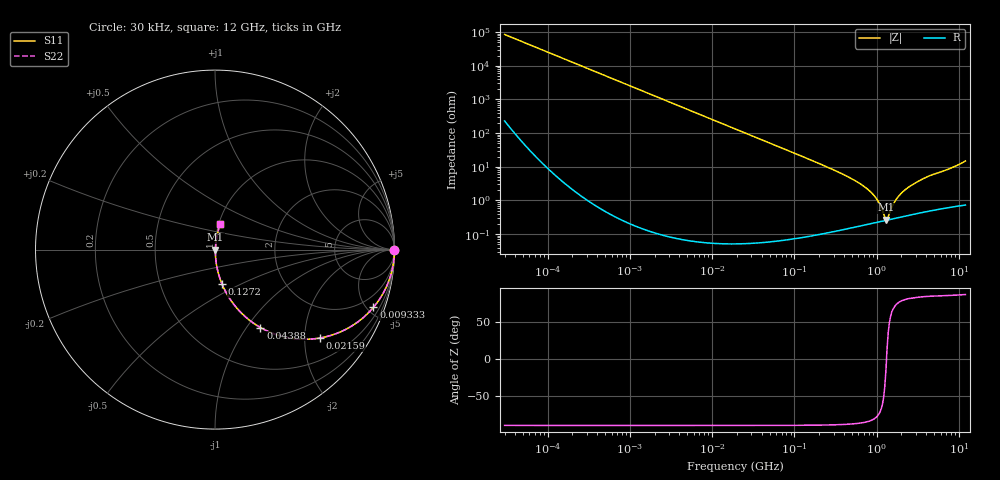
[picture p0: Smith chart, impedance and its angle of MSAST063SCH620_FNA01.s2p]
! MSAST063SCH620_FNA01  S-PARAMETER MODEL  ( Standard Model )
! Model Generated by TAIYO YUDEN Corporation (http://www.ty-top.com)
! Version 1.0
! TAIYO YUDEN Control No. 241122
! Copyright(c) 2024 TAIYO YUDEN CO.,LTD. All Rights Reserved.
! Product Description (link to TY-COMPAS)
! https://ds.yuden.co.jp/TYCOMPAS/or/detail?pn=MSAST063SCH620JFNA01&u=M
! Products Name : Multilayer Ceramic Capacitors
! Characteristics :
!  Capacitance : 62 [pF] , Rated Voltage : 25 [V] , TCC : CH / C0H
!  Case Size : 0.6 x 0.3 / 0.024 x 0.012 [mm/inch] , Thickness : 0.3 / 0.012 [mm/inch]
!  (Conditions: Temperature = 25 [degC] , DC Bias Voltage = 0 [V])
! External Node Assignments :
!  1  o---| |---o  2
! GND o---------o GND
! Frequency Range : 0.03MHz  -  12000MHz  [ 401 STEP ]
# MHZ S RI R 50
! Freq[MHz].  S11 Real  S11 Imag  S21 Real  S21 Imag  S12 Real  S12 Imag  S22 Real  S22 Imag
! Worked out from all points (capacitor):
!   401 points, 30 kHz to 12 GHz, reference 50 ohm
!   read as one part in series: C = 62.2 pF near 32 kHz
!   lowest |Z| = 268 mohm at 1.297 GHz (marker M1)
!   series resonance near 1.319 GHz, so ESL is about 230 pH
!   S11 on the Smith chart (normalised r, x): 30 kHz: open; 9.333 MHz: 1.00, -5.48; 21.59 MHz: 1.00, -2.37; 43.88 MHz: 1.00, -1.16; 127.2 MHz: 1.00, -0.40; 12 GHz: 1.01, +0.30
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0.03  1 -0.00117  4.54e-06 0.00117  4.54e-06 0.00117  1 -0.00117
0.260295  0.9999 -0.0102  0.000105 0.0102  0.000105 0.0102  0.9999 -0.0102
2.258455  0.9923 -0.0876  0.00774 0.0876  0.00774 0.0876  0.9923 -0.0876
5.223303  0.96 -0.196  0.04 0.196  0.04 0.196  0.96 -0.196
9.333359  0.8825 -0.3219  0.1175 0.3219  0.1175 0.3219  0.8825 -0.3219
18.97367  0.645 -0.4783  0.355 0.4783  0.355 0.4783  0.645 -0.4783
21.58598  0.584 -0.4927  0.416 0.4927  0.416 0.4927  0.584 -0.4927
43.88187  0.2535 -0.4345  0.7465 0.4345  0.7465 0.4345  0.2535 -0.4345
71.18072  0.1143 -0.3172  0.8857 0.3172  0.8857 0.3172  0.1143 -0.3172
127.1906  0.0389 -0.1914  0.9611 0.1914  0.9611 0.1914  0.0389 -0.1914
164.6252  0.0237 -0.1492  0.9763 0.1492  0.9763 0.1492  0.0237 -0.1492
419.4166  0.00439 -0.0545  0.9956 0.0545  0.9956 0.0545  0.00439 -0.0545
725.66  0.00248 -0.0245  0.9975 0.0245  0.9975 0.0245  0.00248 -0.0245
1001.808  0.00235 -0.0108  0.9976 0.0108  0.9976 0.0108  0.00235 -0.0108
1296.659  0.00258 -0.000729  0.9974 0.000729  0.9974 0.000729  0.00258 -0.000729
1339.156  0.00262 0.000648  0.9974 -0.000648  0.9974 -0.000648  0.00262 0.000648
1428.372  0.00272 0.00309  0.9973 -0.00309  0.9973 -0.00309  0.00272 0.00309
1573.464  0.0029 0.00671  0.9971 -0.00671  0.9971 -0.00671  0.0029 0.00671
1790.1  0.0032 0.0116  0.9968 -0.0116  0.9968 -0.0116  0.0032 0.0116
2471.32  0.00425 0.0249  0.9958 -0.0249  0.9958 -0.0249  0.00425 0.0249
4140.104  0.00721 0.05  0.9928 -0.05  0.9928 -0.05  0.00721 0.05
12000  0.0285 0.1435  0.9715 -0.1435  0.9715 -0.1435  0.0285 0.1435
